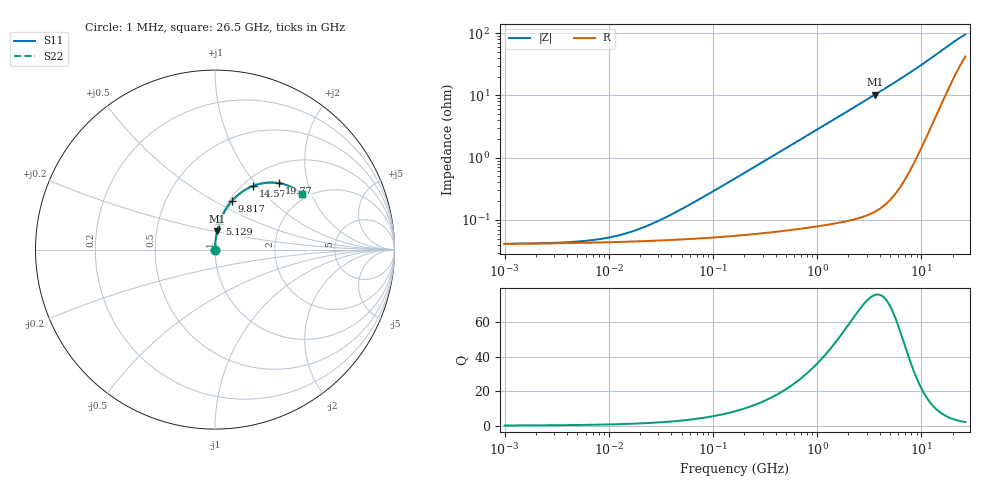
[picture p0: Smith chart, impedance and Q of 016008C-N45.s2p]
# MHz S MA R 50
!Freq  MagS11  AngS11  MagS21  AngS21  MagS12  AngS12  MagS22  AngS22
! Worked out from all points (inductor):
!   801 points, 1 MHz to 26.5 GHz, reference 50 ohm
!   read as one part in series: L = 450 pH near 51.76 MHz
!   highest Q = 75.8 at 3.591 GHz (marker M1), where L = 456 pH
!   S11 on the Smith chart (normalised r, x): 1 MHz: 1.00, +0.00; 5.129 GHz: 1.00, +0.30; 9.817 GHz: 1.03, +0.60; 14.57 GHz: 1.11, +0.95; 19.77 GHz: 1.34, +1.35; 26.5 GHz: 1.84, +1.71
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1  0.000413 3.9  0.9996 -0.0  0.9996 -0.0  0.000413 3.9
2.804488  0.0004277 10.7  0.9996 -0.0  0.9996 -0.0  0.0004277 10.7
5.506729  0.0004558 20.0  0.9996 -0.0  0.9996 -0.0  0.0004558 20.0
8.820004  0.0005023 29.7  0.9996 -0.0  0.9996 -0.0  0.0005023 29.7
13.25558  0.0005811 40.1  0.9996 -0.0  0.9996 -0.0  0.0005811 40.1
19.66978  0.0007177 50.7  0.9995 -0.0  0.9995 -0.0  0.0007177 50.7
29.94045  0.0009662 61.1  0.9995 -0.0  0.9995 -0.0  0.0009662 61.1
58.78931  0.001733 73.4  0.9995 -0.1  0.9995 -0.1  0.001733 73.4
162.7882  0.004634 82.9  0.9994 -0.3  0.9994 -0.3  0.004634 82.9
896.4305  0.02535 86.8  0.9989 -1.5  0.9989 -1.5  0.02535 86.8
1948.898  0.05518 85.8  0.9975 -3.2  0.9975 -3.2  0.05518 85.8
3590.739  0.1021 83.4  0.9934 -5.9  0.9934 -5.9  0.1021 83.4
4873.952  0.1393 81.2  0.9883 -8.0  0.9883 -8.0  0.1393 81.2
5128.584  0.1468 80.7  0.987 -8.4  0.987 -8.4  0.1468 80.7
7418.911  0.2144 76.2  0.9716 -12.4  0.9716 -12.4  0.2144 76.2
9817.014  0.2853 70.9  0.9459 -16.6  0.9459 -16.6  0.2853 70.9
12034.95  0.3487 65.5  0.9122 -20.4  0.9122 -20.4  0.3487 65.5
14567.34  0.4147 58.9  0.8626 -24.3  0.8626 -24.3  0.4147 58.9
17189.29  0.4717 52.2  0.8026 -27.7  0.8026 -27.7  0.4717 52.2
19773.23  0.5149 45.9  0.7407 -30.0  0.7407 -30.0  0.5149 45.9
23631.12  0.5567 37.8  0.6556 -31.3  0.6556 -31.3  0.5567 37.8
26500  0.5743 32.8  0.6035 -31.0  0.6035 -31.0  0.5743 32.8
